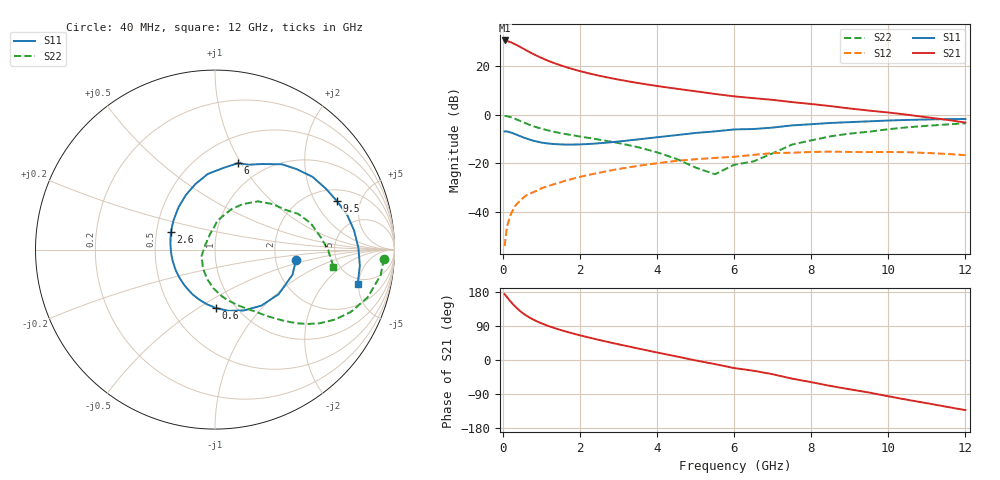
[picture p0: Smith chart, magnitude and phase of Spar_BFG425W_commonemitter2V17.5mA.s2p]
! Filename: 217bfg425.001
! BFG425W Field C1
! V1=8.592E-001V,V2=2.000E+000V, I1=2.449E-004A, I2=1.748E-002A
# GHz  S  MA  R 50
!  S11  S21  S12  S22
!Freq(GHz)  Mag  Ang  Mag  Ang  Mag  Ang  Mag  Ang
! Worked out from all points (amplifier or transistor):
!   44 points, 40 MHz to 12 GHz, reference 50 ohm
!   highest |S21| = 30.5 dB at 40 MHz (marker M1)
!   |S21| within 3 dB of that: start of sweep to 483.1 MHz
!   unconditionally stable (mu >= 1): 1.391 GHz to end of sweep
!   at 700 MHz: K = 0.71, MSG = 29.0 dB, |S12| = -32.4 dB
!   at 2.4 GHz: K = 1.15, MAG = 17.9 dB, |S12| = -24.2 dB
!   at 12 GHz: K = 1.35, MAG = 3.1 dB, |S12| = -16.6 dB
!   S11 on the Smith chart (normalised r, x): 40 MHz: 2.61, -0.37; 600 MHz: 0.82, -0.60; 2.6 GHz: 0.60, +0.12; 6 GHz: 0.76, +0.97; 9.5 GHz: 2.66, +3.09; 12 GHz: 4.26, -4.88
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0.04  0.455 -7.2  33.52 173.9  0.002 78.1  0.942 -3.1
0.1  0.454 -17.9  32.66 166.1  0.005 83.6  0.934 -8.7
0.2  0.433 -35.0  30.8 153.5  0.009 75.9  0.891 -17.4
0.3  0.405 -50.5  28.38 142.6  0.013 71.5  0.833 -24.7
0.4  0.375 -64.7  25.8 133.0  0.016 67.0  0.771 -30.5
0.5  0.349 -77.8  23.33 124.4  0.019 64.0  0.713 -35.1
0.6  0.326 -88.9  21.07 117.4  0.022 62.1  0.661 -38.8
0.7  0.307 -99.0  19.1 111.3  0.024 60.3  0.616 -41.8
0.9  0.279 -116.6  15.92 101.0  0.028 58.2  0.544 -46.4
1  0.268 -124.3  14.64 96.6  0.031 57.4  0.516 -48.4
1.2  0.255 -137.8  12.56 88.8  0.035 56.1  0.471 -51.8
1.6  0.244 -160.5  9.701 76.0  0.044 53.3  0.404 -57.9
2.2  0.25 173.1  7.161 60.1  0.058 47.8  0.337 -67.4
2.6  0.264 158.4  6.072 50.4  0.067 43.5  0.298 -74.2
3.5  0.311 131.0  4.483 30.4  0.089 31.9  0.216 -92.3
4.5  0.381 106.7  3.421 9.4  0.113 17.2  0.124 -122.8
6  0.499 75.0  2.386 -21.3  0.137 -7.3  0.094 106.1
6.5  0.509 68.3  2.19 -28.4  0.15 -10.8  0.11 96.8
8.5  0.678 36.7  1.503 -68.4  0.175 -47.5  0.36 48.3
9.5  0.732 21.6  1.217 -85.9  0.171 -64.0  0.448 29.9
10.5  0.782 7.9  1 -105.1  0.17 -82.4  0.553 15.5
12  0.818 -13.4  0.69 -132.2  0.148 -111.9  0.667 -8.2
